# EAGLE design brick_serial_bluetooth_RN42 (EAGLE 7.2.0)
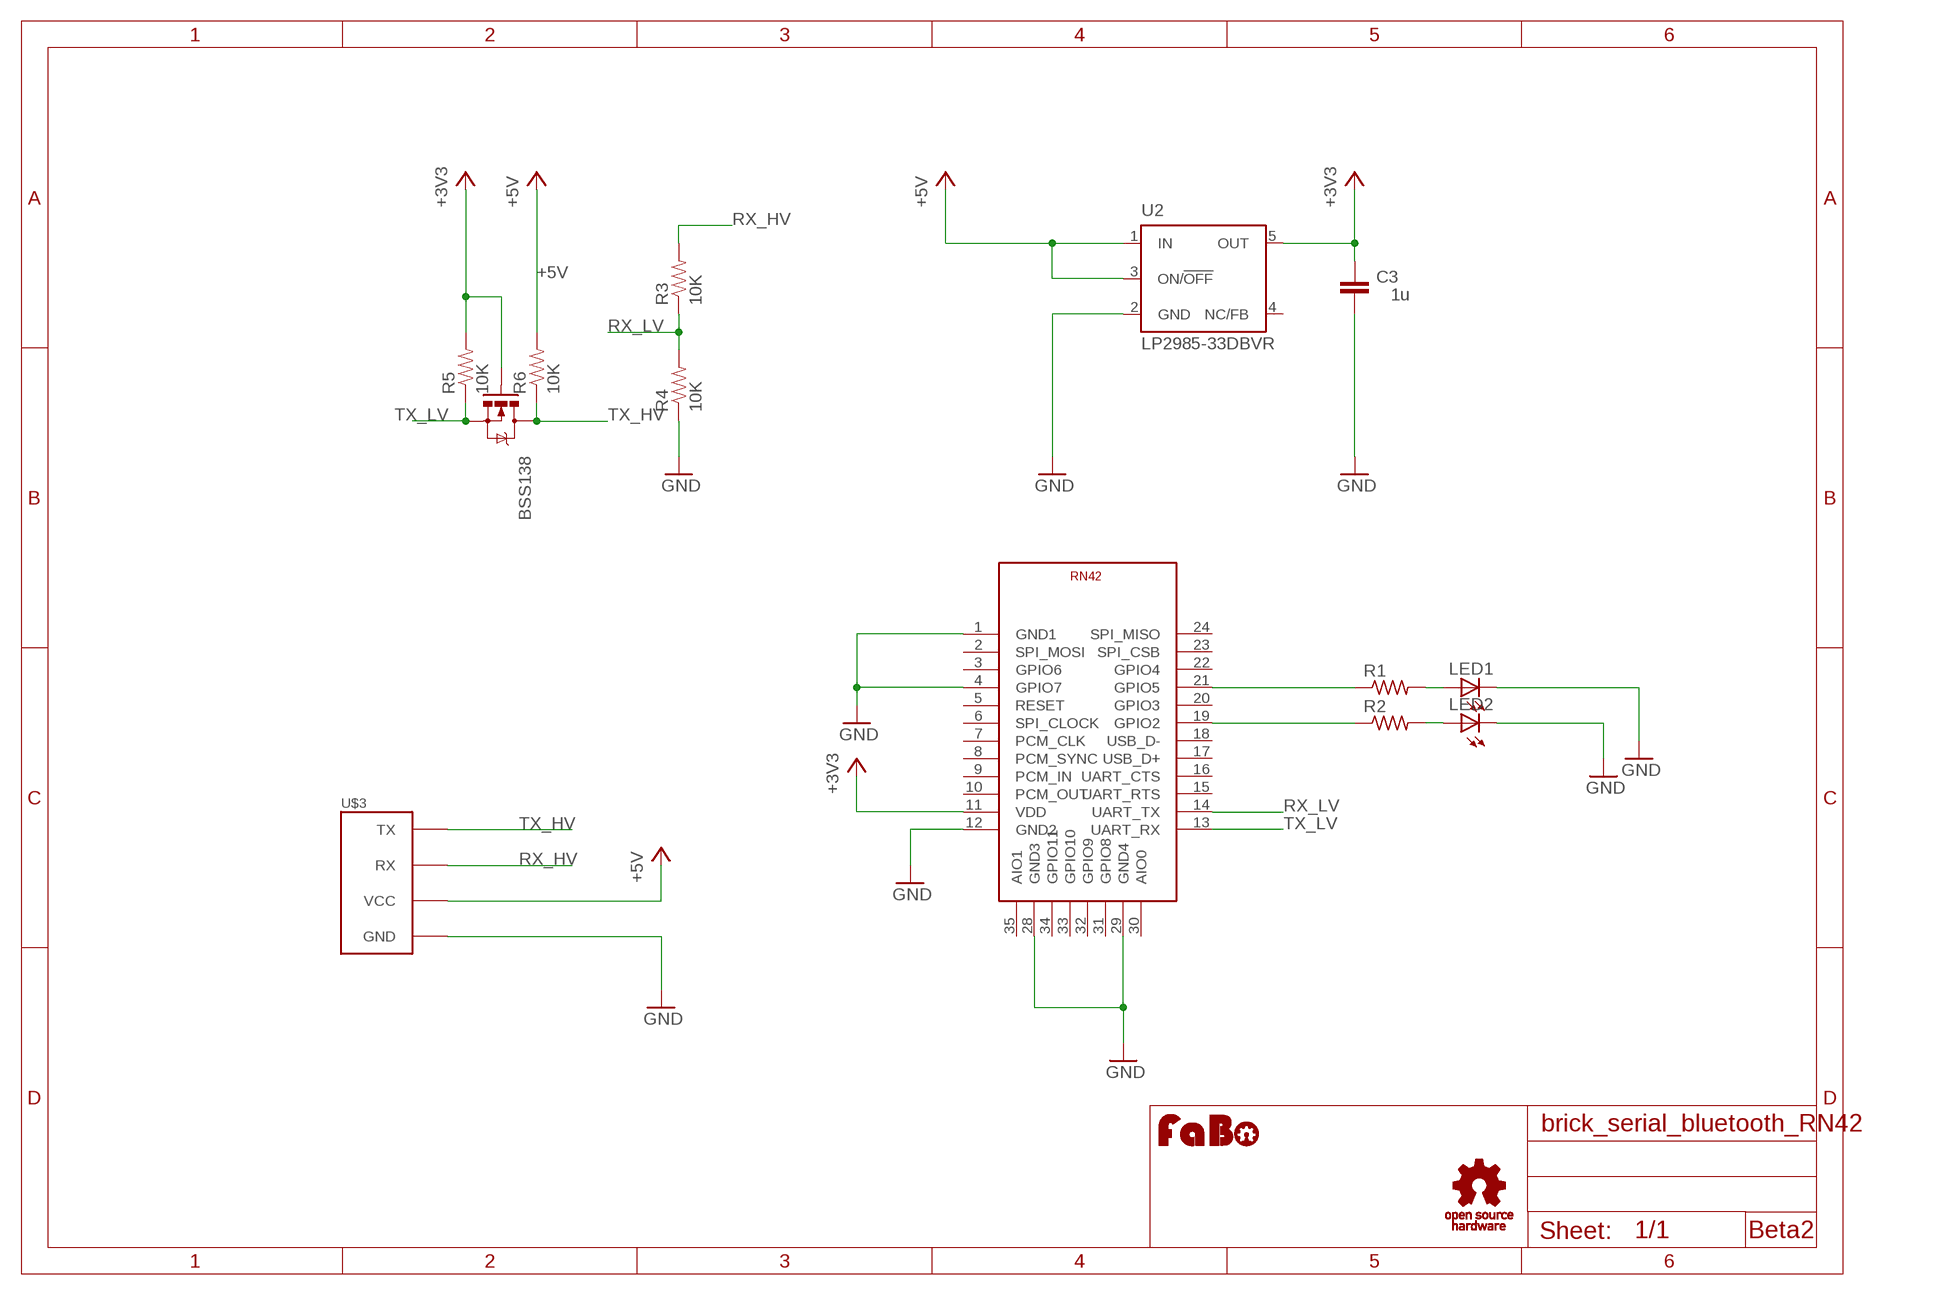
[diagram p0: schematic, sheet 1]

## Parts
BSS138  MOSFET-NCHANNELSMD  [SOT23-3]
C3  1u  C-EU0603-RND  [C0603-ROUND]
LED1  LEDCHIPLED_0603  [CHIPLED_0603]
LED2  LEDCHIPLED_0603  [CHIPLED_0603]
R1  R-US_R0603  [R0603]
R2  R-US_R0603  [R0603]
R3  10K  RESISTOR0603-RES  [0603-RES]
R4  10K  RESISTOR0603-RES  [0603-RES]
R5  10K  RESISTOR0603-RES  [0603-RES]
R6  10K  RESISTOR0603-RES  [0603-RES]
U2  LP2985-33DBVR  LP2985-XXDBVR33  [SOT23-DBV]
U$1  MICROCHIP-RN41  [MICROCHIP-RN42]
U$3  BRICK_SERIAL  [BRICK_SERIAL]
U$4  LOGO_OSHW_T-S  [LOGO_OSHW_T_S]
U$5  LOGO_FABO-S  [LOGO_FABO_S]

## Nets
+3V3: BSS138.1(G) C3.2 R5.2 U2.5(OUT) U$1.11(VDD)
+5V: R6.2 U2.1(IN) U2.3(ON/!OFF) U$3.VCC
GND: C3.1 LED1.C LED2.C R4.1 U2.2(GND) U$1.1(GND1) U$1.4(GPIO7) U$1.12(GND2) U$1.28(GND3) U$1.29(GND4) U$3.GND
N$1: LED1.A R1.2
N$2: R2.1 U$1.19(GPIO2)
N$3: R1.1 U$1.21(GPIO5)
N$4: LED2.A R2.2
RX_HV: R3.2 U$3.RX
RX_LV: R3.1 R4.2 U$1.14(UART_TX)
TX_HV: BSS138.3(D) R6.1 U$3.TX
TX_LV: BSS138.2(S) R5.1 U$1.13(UART_RX)
Unconnected: U2.4(NC/FB) U$1.2(SPI_MOSI) U$1.3(GPIO6) U$1.5(RESET) U$1.6(SPI_CLOCK) U$1.7(PCM_CLK) U$1.8(PCM_SYNC) U$1.9(PCM_IN) U$1.10(PCM_OUT) U$1.15(UART_RTS) U$1.16(UART_CTS) U$1.17(USB_D+) U$1.18(USB_D-) U$1.20(GPIO3) U$1.22(GPIO4) U$1.23(SPI_CSB) U$1.24(SPI_MISO) U$1.30(AIO0) U$1.31(GPIO8) U$1.32(GPIO9) U$1.33(GPIO10) U$1.34(GPIO11) U$1.35(AIO1)

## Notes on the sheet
- Beta2

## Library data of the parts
BSS138 = SparkFun:MOSFET-NCHANNEL
C3 = SmartPrj:C-EU: CAPACITOR, European symbol
LED1 LED2 = adafruit:LED: LED
R1 R2 = adafruit:R-US_: RESISTOR, American symbol
R3-R6 = SparkFun:RESISTOR: Resistor
U2 = SmartPrj:LP2985-XXDBVR: ULTRALOW-POWER 50-mA LOW-DROPOUT LINEAR REGULATORS 50-mA Low-Dropout Regulator Source: http://focus.ti.com/lit/ds/symlink/tps77001.pdf
U$1 = gclueBT:MICROCHIP-RN41
U$3 = gclue:BRICK_SERIAL: FaBo Brick 4pin(SERIAL)
U$4 = gclue:LOGO_OSHW_T
U$5 = FaBo:LOGO_FABO

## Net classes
0 default: clearance 0.254 mm

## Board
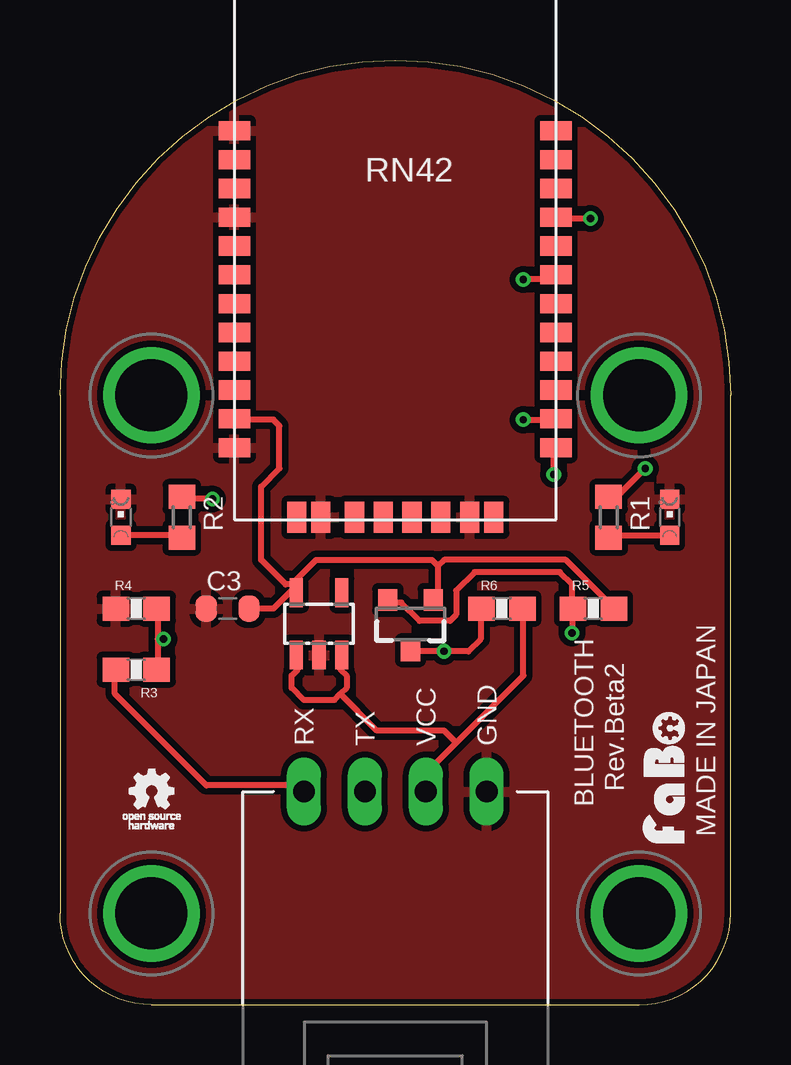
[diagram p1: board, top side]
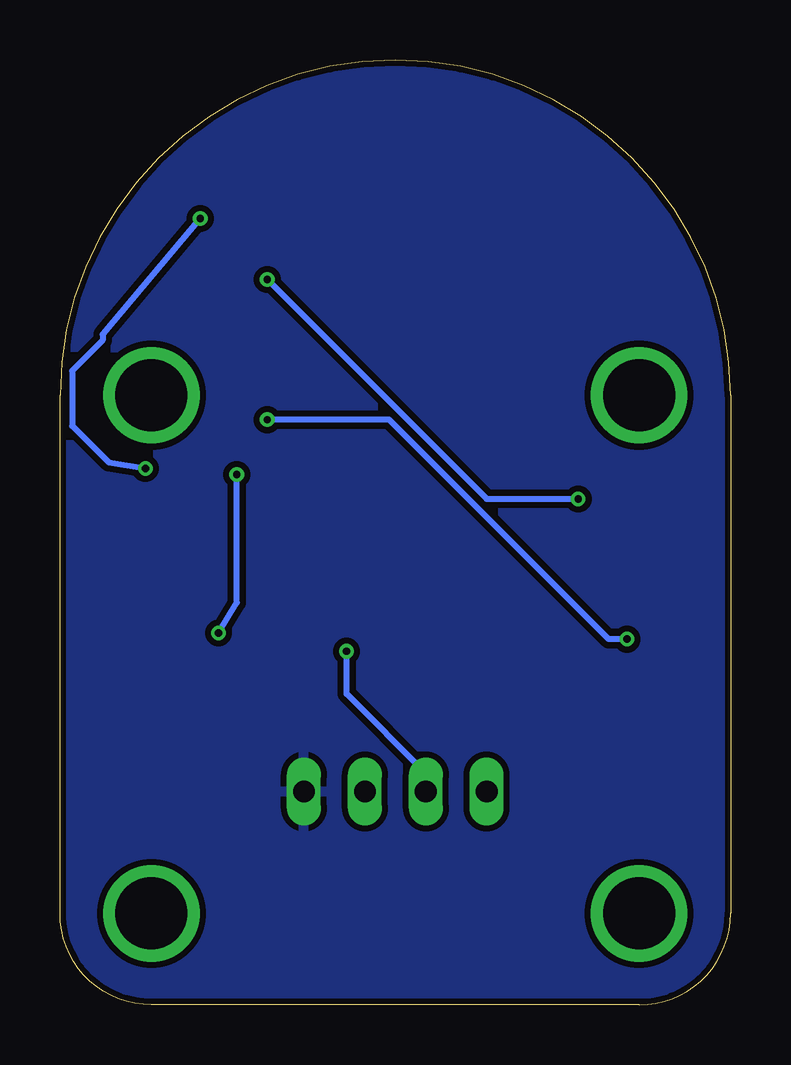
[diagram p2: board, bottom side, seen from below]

Size 27.94 x 39.37 mm. Coordinates in mm from the lower left corner, seen from the top.
Copper layers (1*16): Top 0.035mm / dielectric 1.5mm / Bottom 0.035mm
Design rules "Elecrow_2-layer_eagle_rule": minimum track width 6mil, minimum drill 12mil, track to track 6mil, track to pad 6mil, pad to pad 6mil, via to via 6mil, smd to smd 0mil, copper to edge 10mil, drill to drill 10mil, minimum pad ring 10mil, minimum via ring 6mil, stop-mask expansion 2mil, vias tented up to drill 100mil, thermal gap 10mil

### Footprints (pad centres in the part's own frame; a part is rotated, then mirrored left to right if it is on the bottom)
SOT23-3 = smd 0.8 x 0.9: 1 -0.95,-1; 2 0.95,-1; 3 0,1.1
C0603-ROUND = smd 0.898 x 1.1: 1 -0.889,0; 2 0.889,0
CHIPLED_0603 = smd 0.8 x 0.8: A 0,-0.75; C 0,0.75
R0603 = smd 1 x 1.1: 1 -0.85,0; 2 0.85,0
0603-RES = smd 1.1 x 1: 1 -0.85,0; 2 0.85,0
SOT23-DBV = smd 0.55 x 1.2: 1 -0.95,-1.3; 2 0,-1.3; 3 0.95,-1.3; 4 0.95,1.3; 5 -0.95,1.3
MICROCHIP-RN42 = smd 1.3 x 0.8: 1 -6.7,3.4; 2 -6.7,2.2; 3 -6.7,1; 4 -6.7,-0.2; 5 -6.7,-1.4; 6 -6.7,-2.6; 7 -6.7,-3.8; 8 -6.7,-5; 9 -6.7,-6.2; 10 -6.7,-7.4; 11 -6.7,-8.6; 12 -6.7,-9.8; 13 6.7,-9.8; 14 6.7,-8.6; 15 6.7,-7.4; 16 6.7,-6.2; 17 6.7,-5; 18 6.7,-3.8; 19 6.7,-2.6; 20 6.7,-1.4; 21 6.7,-0.2; 22 6.7,1; 23 6.7,2.2; 24 6.7,3.4 | smd 0.8 x 1.3: 28 3.1,-12.7; 29 -3.1,-12.7; 30 4.1,-12.7; 31 1.9,-12.7; 32 0.7,-12.7; 33 -0.5,-12.7; 34 -1.7,-12.7; 35 -4.1,-12.7
BRICK_SERIAL = drill 0.9 long: GND 3.81,-10.16; RX -3.81,-10.16; TX -1.27,-10.16; VCC 1.27,-10.16 | drill 3 pad 3.81: P$5 -10.16,6.35; P$6 10.16,6.35; P$7 -10.16,-15.24; P$8 10.16,-15.24

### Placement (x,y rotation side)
BSS138  14.61,15.88 180 top
C3  6.99,16.51 0 top
LED1  25.4,20.32 0 top
LED2  2.54,20.32 0 top
R1  22.86,20.32 270 top
R2  5.08,20.32 270 top
R3  3.17,13.97 180 top
R4  3.17,16.51 0 top
R5  22.23,16.51 0 top
R6  18.41,16.51 0 top
U2  10.79,15.88 0 top
U$1  13.97,33.02 0 top
U$3  13.97,19.05 0 top
U$4  3.81,8.89 0 top
U$5  26.04,9.53 90 top

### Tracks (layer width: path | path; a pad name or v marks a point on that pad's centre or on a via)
+3V3
  Top 0.254: 15.75,18.29 15.75,17.02 BSS138.1 | 15.75,18.29 16,18.54 21.08,18.54 23.11,16.51 R5.2 | C3.2 8.89,16.51 9.65,17.27 U2.5 | 9.65,17.53 9.91,17.53 9.91,17.27 U2.5 | 9.65,17.53 9.4,17.53 8.38,18.54 8.38,21.59 9.14,22.35 9.14,24.13 8.89,24.38 7.37,24.38 U$1.11 | 15.75,18.29 15.49,18.54 10.67,18.54 9.65,17.53 | 9.65,17.53 U2.5
+5V
  Top 0.254: 11.68,12.95 11.94,13.21 11.94,13.72 11.68,13.97 11.68,14.48 U2.3 | 11.68,12.95 11.43,12.7 10.16,12.7 9.65,13.21 9.65,13.72 9.91,13.97 9.91,14.48 U2.1 | 16.51,10.92 15.24,9.65 U$3.VCC | 16.51,10.92 19.3,13.72 19.3,16.51 R6.2 | 11.68,12.95 13.21,11.43 16,11.43 16.51,10.92
GND
  pour Bottom: -1.27,-1.27 29.21,-1.27 29.21,40.64 -1.27,40.64
  pour Top: -1.27,-1.27 29.21,-1.27 29.21,40.64 -1.27,40.64
N$1
  Top 0.254: LED1.A 25.4,19.56 22.86,19.56 R1.2
N$2  (via drill 0.3)
  Top 0.254: v6.35,21.08 5.08,21.08 R2.1 | v19.3,30.23 20.57,30.23 U$1.19
  Bottom 0.254: v6.35,21.08 10.16,21.08 v19.3,30.23
N$3  (via drill 0.3)
  Top 0.254: v24.38,22.35 23.37,21.34 22.86,21.34 R1.1 | v22.1,32.77 20.83,32.77 U$1.21
  Bottom 0.254: v24.38,22.35 25.91,22.61 27.43,24.13 27.43,26.42 26.16,27.69 26.16,27.94 v22.1,32.77
N$4
  Top 0.254: LED2.A 2.54,19.56 5.08,19.56 R2.2
RX_HV
  Top 0.254: U$3.RX 9.91,9.14 6.1,9.14 2.29,12.95 2.29,13.97 R3.2
RX_LV  (via drill 0.3)
  Top 0.254: 4.06,15.24 4.06,16.51 R4.2 | 4.06,15.24 4.06,13.97 R3.1 | v19.3,24.38 20.57,24.38 U$1.14 | 4.06,15.24 v4.32,15.24
  Bottom 0.254: v19.3,24.38 14.22,24.38 5.08,15.24 v4.32,15.24
TX_HV  (via drill 0.3)
  Top 0.254: BSS138.3 14.73,14.73 v16,14.73 17.02,14.73 17.53,15.24 17.53,16.51 R6.1
  Bottom 0.254: v16,14.73 16,12.95 12.7,9.65 U$3.TX
TX_LV  (via drill 0.3)
  Top 0.254: 21.34,16.51 21.34,17.53 20.83,18.03 17.27,18.03 16.51,17.27 16.51,16.26 16.26,16 14.99,16 14.22,16.76 13.72,16.76 BSS138.2 | v20.57,22.1 20.57,23.11 U$1.13 | 21.34,16.51 v21.34,15.49 | 21.34,16.51 R5.1
  Bottom 0.254: v20.57,22.1 20.57,16.76 v21.34,15.49

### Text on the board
tPlace: RN42 | MADE IN JAPAN | Rev.Beta2 | BLUETOOTH

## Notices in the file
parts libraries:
SparkFun: Licensing: CC v3.0 Share-Alike You are welcome to use this library for commercial purposes.
